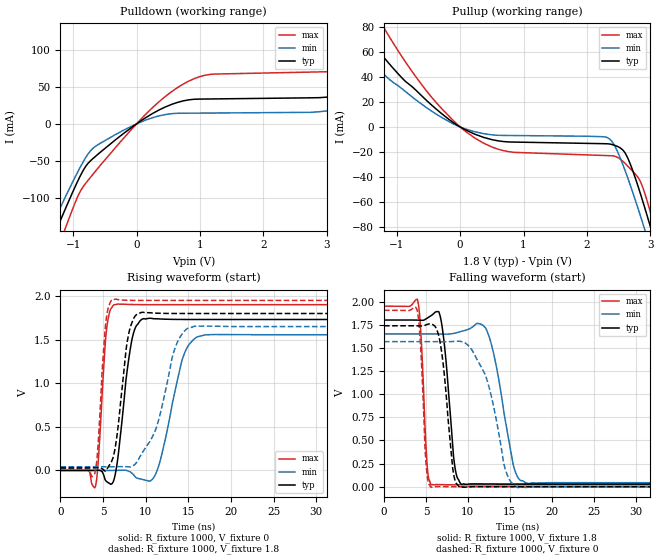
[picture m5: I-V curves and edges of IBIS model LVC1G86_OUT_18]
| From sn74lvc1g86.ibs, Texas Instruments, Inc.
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[Model]   LVC1G86_OUT_18
Model_type  Output
Vref =   0
Rref =   1000
Cref =   30p
Vmeas =   0.9
| variable   typ   min   max
C_comp   9.73pF   6.40pF   16.46pF
| C_pullup   8.77pF   6.40pF   9.60pF
| C_pulldown   10.70pF   6.77pF   16.46pF
[Temperature Range]   40   100   -40
| Ambient temperature   25   85   -40
[Voltage range]   1.8   1.65   1.95
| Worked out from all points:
|   slope of the pulldown table from 0 to 0.27 V, typ, clamps not added: 18.2 ohm
|   slope of the pullup table from 0 to 0.27 V, typ, clamps not added: 41.4 ohm
|   rising waveform, R_fixture 1000, V_fixture 0: 20-80 % time 1.21ns typ, 2.02ns min, 697ps max; typ from 0 V to 1.73 V
|   falling waveform, R_fixture 1000, V_fixture 1.8: 20-80 % time 944ps typ, 1.83ns min, 570ps max; typ from 1.8 V to 0.029 V
|   rising waveform, R_fixture 1000, V_fixture 1.8: 20-80 % time 1.18ns typ, 2.53ns min, 711ps max; typ from 0.029 V to 1.8 V
|   falling waveform, R_fixture 1000, V_fixture 0: 20-80 % time 1.07ns typ, 2.35ns min, 560ps max; typ from 1.74 V to 0 V
[Pulldown]
| LVC1G86_OUT_18
|   Voltage   I(typ)   I(min)   I(max)
-5V       -903.9mA   -822.2mA   -1.038A
-1.47V    -185.3mA   -162.1mA   -223mA
-1.265V   -143.5mA   -124.5mA   -174.4mA
-1.11V    -112.3mA   -96.52mA   -138.1mA
-650mV    -44.1mA    -30.47mA   -64.2mA
730mV     30.93mA    14.37mA    53.46mA
3.33V     41.21mA    22.81mA    73.44mA
4.21V     64.59mA    16.31mA    107.6mA
4.445V    38.62mA    16.42mA    120.3mA
4.7V      37.61mA    16.54mA    130.5mA
5.1V      37.87mA    16.73mA    75.56mA
10V       42.22mA    18.93mA    82.87mA
[Pullup]
| LVC1G86_OUT_18
|   Voltage   I(typ)   I(min)   I(max)
-5V       356.3mA    216.8mA    497.8mA
-2.1V     116mA      89.72mA    163.3mA
-1.66V    84.87mA    65.06mA    120.2mA
-1.285V   60.52mA    45.86mA    86.2mA
-385mV    14.58mA    10.47mA    19.89mA
370mV     -8.345mA   -5.376mA   -12.96mA
2.35V     -13.59mA   -9.345mA   -22.94mA
2.605V    -21.18mA   -35.46mA   -29.37mA
2.91V     -64.47mA   -81.84mA   -52.86mA
3.055V    -89.29mA   -105.6mA   -78.27mA
3.155V    -107mA     -122.3mA   -97.29mA
10V       -1.474A    -1.396A    -1.611A
[Ramp]
| LVC1G86_OUT_18
| variable   typ   min   max
dV/dt_r   1.14/1.37E-09   1.01/2.22E-09   1.26/7.73E-10
dV/dt_f   1.12/1.03E-09   1.03/2.03E-09   1.20/6.34E-10
R_load = 1000
[Rising Waveform]
| LVC1G86_OUT_18
R_fixture =   1000
C_fixture =   0
L_fixture =   0
V_fixture =   0
V_fixture_min = 0
V_fixture_max = 0
|   Time   V(typ)   V(min)   V(max)
0s        120.1pV    8.639nV    662.4pV
4.095ns   820.7uV    -18.75uV   -184.6mV
5.375ns   -124.6mV   -34.07uV   1.589V
6.31ns    -94.11mV   437.1uV    1.901V
8.3ns     1.458V     -24.61mV   1.903V
9.62ns    1.737V     -103mV     1.901V
11.3ns    1.739V     -8.788mV   1.901V
14.22ns   1.732V     1.252V     1.901V
16.06ns   1.731V     1.533V     1.901V
50ns      1.731V     1.556V     1.901V
[Falling Waveform]
| LVC1G86_OUT_18
R_fixture =   1000
C_fixture =   0
L_fixture =   0
V_fixture =   1.8
V_fixture_min = 1.65
V_fixture_max = 1.95
|   Time   V(typ)   V(min)   V(max)
0s        1.8V       1.65V      1.95V
3.995ns   1.799V     1.65V      2.017V
5.145ns   1.82V      1.65V      228.3mV
5.655ns   1.85V      1.65V      18.61mV
6.835ns   1.78V      1.649V     22.69mV
8.335ns   289.2mV    1.656V     20.54mV
9.235ns   26.01mV    1.678V     20.54mV
12.28ns   29.61mV    1.683V     20.73mV
16.91ns   29.14mV    40.82mV    20.74mV
50ns      29.16mV    42.33mV    20.74mV
[Rising Waveform]
| LVC1G86_OUT_18
R_fixture =   1000
C_fixture =   0
L_fixture =   0
V_fixture =   1.8
V_fixture_min = 1.65
V_fixture_max = 1.95
|   Time   V(typ)   V(min)   V(max)
0s        29.14mV    42.29mV    20.74mV
4.035ns   29.66mV    42.28mV    -31.33mV
4.385ns   30.98mV    42.29mV    255.6mV
5.275ns   -6.253mV   42.29mV    1.655V
6.06ns    118.3mV    42.37mV    1.957V
7.95ns    1.542V     42.07mV    1.951V
9.39ns    1.81V      168.1mV    1.95V
13.53ns   1.8V       1.428V     1.95V
15.03ns   1.8V       1.634V     1.95V
50ns      1.8V       1.65V      1.95V
[Falling Waveform]
| LVC1G86_OUT_18
R_fixture =   1000
C_fixture =   0
L_fixture =   0
V_fixture =   0
V_fixture_min = 0
V_fixture_max = 0
|   Time   V(typ)   V(min)   V(max)
0s        1.738V     1.567V     1.905V
3.965ns   1.738V     1.567V     1.903V
5.02ns    1.749V     1.567V     239.1mV
5.62ns    1.757V     1.567V     -6.537mV
6.7ns     1.553V     1.566V     1.015mV
8.19ns    199mV      1.569V     -192.9uV
9.055ns   -8.473mV   1.57V      -209.8uV
12.08ns   100.6uV    1.209V     -60.92nV
15.89ns   8.461uV    -7.399mV   7.478uV
50ns      12.79uV    32.59uV    4.88uV
